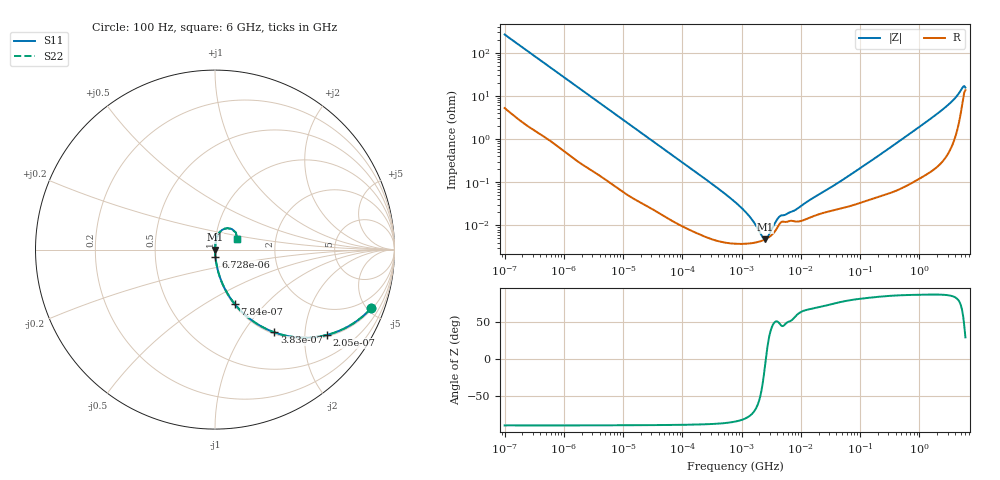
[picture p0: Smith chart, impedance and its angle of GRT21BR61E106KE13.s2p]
!Murata Part Number: GRT21BR61E106KE13
!These Parameters are Measured in Series Mode Connection
!Data Generated on Jun 19, 2026
!  o--ll--o
!Port1  Port2
!  o------o
!Operation Temp=25[degC], DC Bias Voltage=0[V]
!Freq. Start=100[Hz] Stop=6[GHz] 401[Steps]
# Hz S RI R 50
!Freq.(Hz) S11(Real) S11(Imag) S21(Real) S21(Imag) S12(Real) S12(Imag) S22(Real) S22(Imag)
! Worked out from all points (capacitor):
!   401 points, 100 Hz to 6 GHz, reference 50 ohm
!   read as one part in series: C = 6.02 uF near 109 Hz
!   lowest |Z| = 4.77 mohm at 2.481 MHz (marker M1)
!   series resonance near 2.567 MHz, so ESL is about 640 pH
!   S11 on the Smith chart (normalised r, x): 100 Hz: 1.10, -5.26; 205 Hz: 1.05, -2.59; 383 Hz: 1.03, -1.39; 784 Hz: 1.01, -0.69; 6.728 kHz: 1.00, -0.08; 6 GHz: 1.27, +0.15
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100  0.8689 -0.3278  0.1311 0.3278  0.1311 0.3278  0.8689 -0.3278
137  0.7841 -0.4021  0.2159 0.4021  0.2159 0.4021  0.7841 -0.4021
205  0.6245 -0.4752  0.3755 0.4752  0.3755 0.4752  0.6245 -0.4752
383  0.33 -0.4607  0.67 0.4607  0.67 0.4607  0.33 -0.4607
784  0.1104 -0.3038  0.8896 0.3038  0.8896 0.3038  0.1104 -0.3038
2008  0.0205 -0.1326  0.9795 0.1326  0.9795 0.1326  0.0205 -0.1326
6728  0.00255 -0.041  0.9975 0.041  0.9975 0.041  0.00255 -0.041
40335  0.000242 -0.00703  0.9998 0.00703  0.9998 0.00703  0.000242 -0.00703
774597  3.76e-05 -0.000346  1 0.000346  1 0.000346  3.76e-05 -0.000346
1159002  3.75e-05 -0.000203  1 0.000203  1 0.000203  3.75e-05 -0.000203
1734173  4.01e-05 -9.31e-05  1 9.31e-05  1 9.31e-05  4.01e-05 -9.31e-05
2481164  4.7e-05 -7.9e-06  1 7.9e-06  1 7.9e-06  4.7e-05 -7.9e-06
3394479  6.41e-05 6.76e-05  0.9999 -6.76e-05  0.9999 -6.76e-05  6.41e-05 6.76e-05
4440638  0.000111 0.00012  0.9999 -0.00012  0.9999 -0.00012  0.000111 0.00012
7947587  0.000123 0.000187  0.9999 -0.000187  0.9999 -0.000187  0.000123 0.000187
1.555665e7  0.000159 0.000387  0.9998 -0.000387  0.9998 -0.000387  0.000159 0.000387
4.983056e7  0.00025 0.00108  0.9998 -0.00108  0.9998 -0.00108  0.00025 0.00108
3.124326e8  0.000588 0.0061  0.9994 -0.0061  0.9994 -0.0061  0.000588 0.0061
1.712697e9  0.00295 0.0324  0.9971 -0.0324  0.9971 -0.0324  0.00295 0.0324
3.505958e9  0.0117 0.0713  0.9883 -0.0713  0.9883 -0.0713  0.0117 0.0713
5.245841e9  0.07 0.1195  0.93 -0.1195  0.93 -0.1195  0.07 0.1195
6e9  0.1228 0.0584  0.8772 -0.0584  0.8772 -0.0584  0.1228 0.0584
